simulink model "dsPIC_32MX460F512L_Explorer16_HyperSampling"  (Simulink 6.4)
settings: Solver=FixedStepDiscrete  StartTime=0.0  StopTime=10.0  FixedStep=.001  RelTol=1e-3
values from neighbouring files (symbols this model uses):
  OCmax = 9599    [RC_experiment.m]
undefined symbols (not defined in the file or in its folder): bits, Buffer, characters, contain, full, is, OC_HW, PWM, Receive, Timer3, When
libraries: dsPICdrivers x7, simulink x2

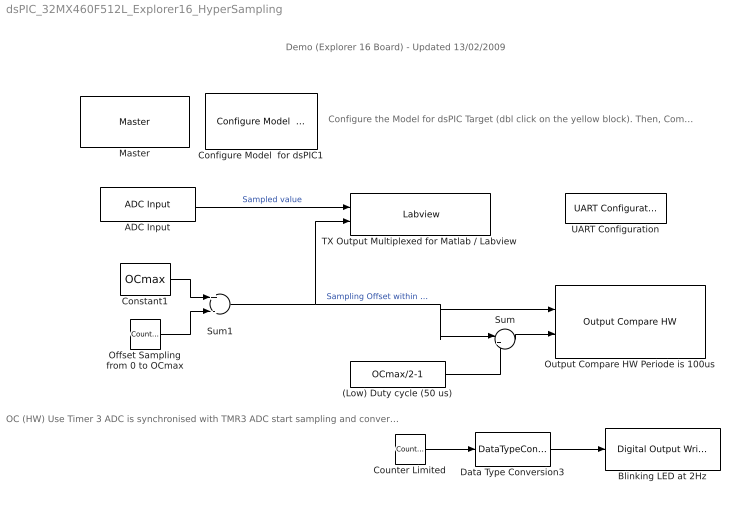
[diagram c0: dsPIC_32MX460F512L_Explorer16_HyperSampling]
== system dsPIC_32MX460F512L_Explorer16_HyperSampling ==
  note: Demo (Explorer 16 Board) - Updated 13/02/2009
  note: Configure the Model for dsPIC Target (dbl click on the yellow block). Then, Compile using the incremental build icon (second icon on right of the simulation mode (Normal))
  note: OC (HW) Use Timer 3 ADC is synchronised with TMR3 ADC start sampling and converting when TMR3 = OCmax (=PR3)
  (Low) Duty cycle (50 us) : Constant  Value=OCmax/2-1  OutDataTypeMode=uint16  OutDataType=sfix(16)  OutScaling=2^0
  ADC Input : dsPICdrivers/Peripheral I//O/ADC Input  Tag=dsPIC_ADC  Priority=5  ADC_TYPE=10 bits  ADC_MODE=Continuous sampling & get last channel value  NbrSampleStep=1  VoltRefpopup="AVdd  -  AVss"  OutFormatBitspopup=0000 00dd dddd dddd : Integer  InterruptPriority=6  ANCHANNELS=5  MaxName=ANmax = 1024  Rin=5e6  ADCS=29  SAMC=31  Temperature=25  DMAChannel=0  SampleTime=.001  Status="OK  |  Tsmp=4.844e-006 |  T/Channel=6.719e-006 |  Tall=6.719e-006"  SSRC=Timer3 (OC_HW PWM)
  Blinking LED at 2Hz : dsPICdrivers/Digital I//O/Digital Output Write  Tag=dsPIC_Digital_Output  Priority=5  PORT=A  Simultaneous=off  OrderingInOutPopup=None
  Configure Model  for dsPIC1 : dsPICdrivers/Simulink Configuration/Configure Model  for dsPIC
  Constant1 : Constant  Value=OCmax  OutDataTypeMode=uint16  OutDataType=sfix(16)  OutScaling=2^0
  Counter Limited : simulink/Sources/Counter Limited  SystemSampleTime=-1  uplimit=1  tsamp=.25
  Data Type Conversion3 : DataTypeConversion  OutDataTypeMode=boolean  OutDataType=sfix(16)  OutScaling=2^0
  Master : dsPICdrivers/Master  Tag=dsPIC_MASTER  Priority=1  TimeStepType=Timer1  picType=32MX460F512L  fcy=96000000  Quartz_33f=8e6  PLLActive_33f=on  fcyDesired_33f=96e6  tmr1="[8  11999  0]"  tmr1Info="Time Step : 0.001  ;   Error : 0%  PR1=11999"  tmr2345="[0  1  0  0]"  tmr2345cfg=[-1 -1 -1 -1]  IOautoConf=on  typePort="[ 10   0   0   0   0   0   0   0   0   0   0   0   0   0   0   0   0   0   0   0   0   8   0   0   0   0   0   0   0   0   0   0   0   0   0   0   0   0   0   0   0   0   0   0   0   0   0   0  24   0   0   0   0   0   0   0   0   0   0   0   0   0   0   0   0   0   0   0   0   0   0   0   0   0   0   0   0   0   0   0   0   0   0   0   4   5   0   0   0   0   0   0   0   0   0   0   0   0   0   0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"  TRIS="[ 65534  65535  65535  65534  65535  65535  65535 ]"  ADPCFG=0  MasterBusyPort=None  MasterOverloadPort=None  FOSC=Quartz (XT - HS)  ClockSwitchMonitor=Both disabled  TempProtection_33f=TEMP_ON  FPBOR=<empty>  PWRT=disable  MCLR=<empty>  PowerSave=off  OverrideFcy=off  NewFcy=1e6  PR2345="[65535   9599  65535  65535]"
  Offset Sampling from 0 to OCmax : simulink/Sources/Counter Limited  SystemSampleTime=-1  uplimit=OCmax  tsamp=.001
  Output Compare HW Periode is 100us : dsPICdrivers/Peripheral I//O/Output Compare HW  Tag=dsPIC_OC_HW_out  Priority=5  OC_Mode=PWM Time Set-Reset (glitch possible)  Timer=3  CHANNEL=[1 ]  Channel_UP_Down_Periode=[16]  PeriodeInput=off  MaxChannel=0.0001  MaxName=' OCmax '  Precision=[13.2288]  Status=OK  SafeMarge=[0]  PortLetter=[68]  PortNumber=[0]  MaxValues=[9599]  NPORTS=2
  Sum : Sum  Inputs=|++  OutDataType=sfix(16)  OutScaling=2^0
  Sum1 : Sum  Inputs=+-  OutDataType=sfix(16)  OutScaling=2^0
  TX Output Multiplexed for Matlab / Labview : dsPICdrivers/Serial PORT/TX Output Multiplexed for Matlab // Labview  Tag=dsPIC_TX_Multiplexed  Priority=5  UART=2  CleverSpreadingChk=on  CleverSpreading=1  CHANNEL=[0 1]  CHANNELBLOCKED=[]  CHANNELBLOCKED_BITEWISE=0  Status=OK
  UART Configuration : dsPICdrivers/Serial PORT/UART Configuration  Tag=dsPIC_config_UART  Priority=2  UART=2  proposed_BAUD=115200  ALT_TX_RX=on  InterruptTxWhen=When Transmit Buffer is empty  TXInterruptPri=1  TxBufferSize=32  TXEN=on  InterruptRxWhen=When Receive Buffer is full (contain 4 characters)  RXInterruptPri=2  RxBufferSize=32  BAUD=115200  UxBRG=51  Info="UxBRG = 51   ||  Real Baud : 115385   ||  % error : 0.16026  ||  max 11.5385 Bytes / Step"  RealBaud=0
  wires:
  Counter Limited/1 -> Data Type Conversion3/1
  ADC Input/1 -> TX Output Multiplexed for Matlab / Labview/1  "Sampled value"
  (Low) Duty cycle (50 us)/1 -> Sum/2
  Sum/1 -> Output Compare HW Periode is 100us/2
  Sum1/1 -> Output Compare HW Periode is 100us/1, Sum/1, TX Output Multiplexed for Matlab / Labview/2  "Sampling Offset within PWM"
  Constant1/1 -> Sum1/1
  Offset Sampling from 0 to OCmax/1 -> Sum1/2
  Data Type Conversion3/1 -> Blinking LED at 2Hz/1
